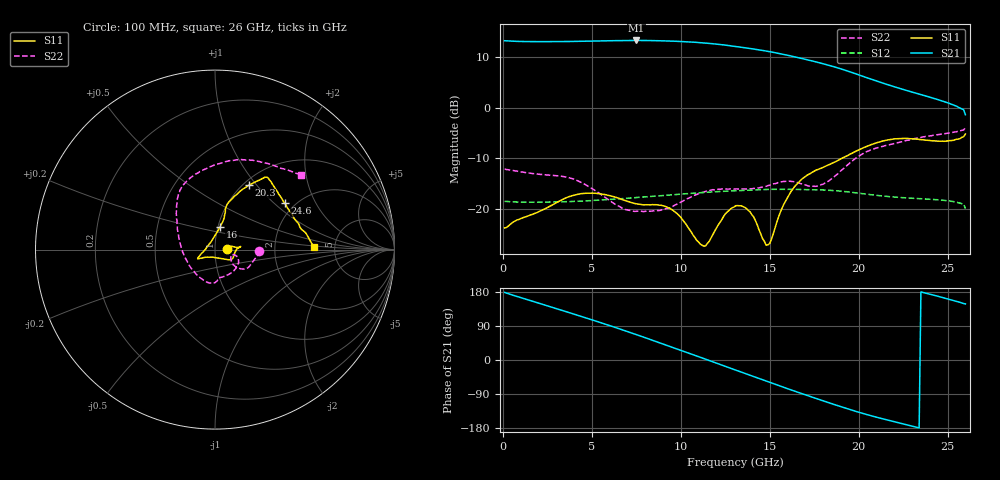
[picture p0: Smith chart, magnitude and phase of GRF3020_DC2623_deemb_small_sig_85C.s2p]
!Keysight Technologies,N5245B,MY56052315,A.20.20.05
!Date: Tuesday, July 28, 2026 13:42:05
!Correction: S11(C  2-Port  )
!S21(C  2-Port  )
!S12(C  2-Port  )
!S22(C  2-Port  )
!S2P File: Measurements: S11, S21, S12, S22:
# Hz S  dB  R 50
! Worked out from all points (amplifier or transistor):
!   260 points, 100 MHz to 26 GHz, reference 50 ohm
!   highest |S21| = 13.2 dB at 7.5 GHz (marker M1)
!   |S21| within 3 dB of that: start of sweep to 16.12 GHz
!   unconditionally stable (mu >= 1): start of sweep to end of sweep
!   at 4.4 GHz: K = 1.16, MAG = 13.3 dB, |S12| = -18.4 dB
!   at 13.1 GHz: K = 1.10, MAG = 12.3 dB, |S12| = -16.4 dB
!   at 26 GHz: K = 2.52, MAG = 2.4 dB, |S12| = -19.9 dB
!   S11 on the Smith chart (normalised r, x): 100 MHz: 1.14, +0.01; 16 GHz: 1.02, +0.26; 20.3 GHz: 1.06, +0.91; 24.6 GHz: 1.77, +1.17; 26 GHz: 3.43, +0.16
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1e8  -23.69 2.7  13.16 178.3  -18.46 -0.8  -12.11 -1.7
1.3e9  -21.49 12.1  12.99 160.4  -18.63 -7.8  -12.81 -12.9
2.3e9  -20.04 10.1  12.98 145.9  -18.62 -13.1  -13.22 -20.3
3.4e9  -18.02 5.3  13.00 129.9  -18.54 -19.1  -13.58 -28.9
4.5e9  -16.91 6.2  13.05 113.7  -18.40 -25.1  -14.90 -36.6
5.3e9  -16.90 6.9  13.10 101.6  -18.26 -29.7  -16.58 -39.9
6.1e9  -17.43 5.5  13.16 89.3  -18.07 -34.4  -18.55 -37.3
7.5e9  -18.94 -6.7  13.21 67.1  -17.71 -43.5  -20.42 -20.9
8.8e9  -19.21 -27.3  13.15 45.8  -17.37 -52.6  -20.27 -17.9
9.9e9  -21.22 -39.5  13.03 27.6  -17.08 -60.8  -18.82 -15.6
1.1e10  -26.45 -77.7  12.82 9.0  -16.79 -69.5  -16.94 -23.0
1.2e10  -23.75 -139.1  12.49 -8.1  -16.56 -77.9  -16.10 -41.6
1.31e10  -19.31 -151.2  12.03 -26.8  -16.37 -87.4  -16.00 -69.3
1.39e10  -20.54 -157.7  11.63 -40.3  -16.25 -94.5  -15.98 -80.7
1.48e10  -27.10 150.8  11.13 -55.5  -16.12 -102.8  -15.50 -84.3
1.6e10  -17.70 77.3  10.30 -75.6  -16.08 -114.4  -14.54 -97.3
1.74e10  -12.71 75.5  9.16 -98.2  -16.16 -127.8  -15.47 -142.7
1.88e10  -10.47 71.3  7.84 -120.2  -16.39 -141.6  -13.12 157.4
2.03e10  -7.85 62.4  6.07 -141.9  -16.99 -155.3  -8.94 125.6
2.17e10  -6.33 55.8  4.43 -159.3  -17.52 -166.1  -7.34 106.0
2.46e10  -6.63 33.6  1.40 166.4  -18.21 170.7  -5.26 64.6
2.6e10  -5.20 1.7  -1.41 148.0  -19.89 156.5  -3.97 41.0
